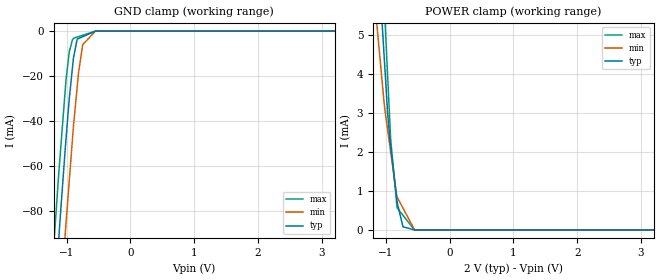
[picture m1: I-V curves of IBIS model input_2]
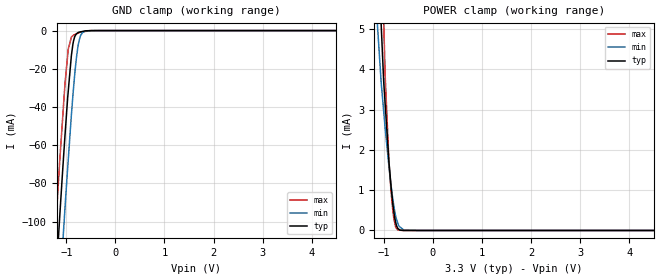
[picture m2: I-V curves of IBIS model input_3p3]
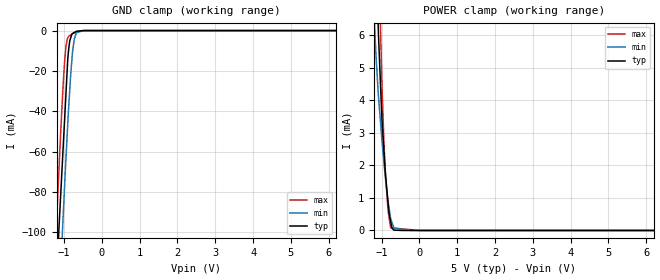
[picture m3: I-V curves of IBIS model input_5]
|Texas Instruments Incorporated
|16-Bit, Quad Channel, Ultralow Glitch, Voltage Output Digital to
|Analog Converter
|Marketing part#   Digital Voltage Range   Package-type   #pins
| DAC8555IPW   1.8V - 5.5V   TSSOP   16
| DAC8555IPWG4   1.8V - 5.5V   TSSOP   16
| DAC8555IPWR   1.8V - 5.5V   TSSOP   16
| DAC8555IPWRG4   1.8V - 5.5V   TSSOP   16
[IBIS Ver]   3.2
[File name]   dac8555.ibs
|SIMDE Ver   V3.0 - 201101 - RHL4 - Build 457
[File Rev]   1.0
[Date]   7/05/2011
[Source]
| Texas Instruments Incorporated.
| Analog-eLab Design Center, HPA
| 12500 TI Blvd
| Dallas, TX -75243
| e-mail: elab_ibis@list.ti.com
[Notes]   Revision History:
| Rev 1.0: 7/05/2011
| - Initial version of the model
| - Model generated from simulations in TISPICE
| - Model matched to SPICE simulation
| - C_comp although listed in numerical order of value are
|   obtained from varying PVT conditions. For PVT conditions for
|   each specific value refer the buffer description under
|   respective [Model]. IBIS model user is responsible for using
|   appropriate C_comp to simulate for Signal Integrity.
| - Model names with a trailing _2 contains the model for
|   2V [1.8V and 2.2V].
| - Model names with a trailing _3p3 contains the model for
|   3.3V [3.0V and 3.6V]. Model names with a trailing _5 contains
|   the model for 5.0V [4.5V and 5.5V].
[Disclaimer]
| This model is designed as an aid for customers of Texas Instruments.
| TI and its licensors and suppliers make no warranties, either expressed
| or implied, with respect to this  model, including the warranties of
| merchantability or fitness for a particular purpose. The model is
| provided solely on an "as is" basis. The entire risk as to its quality
| and performance is with the customer.
[Copyright]
 (C) Copyright 2011 Texas Instruments Incorporated.All rights reserved.
|   DAC8555
[Component]   DAC8555
[Manufacturer]   TI
[Package]   |16 TSSOP - PW package
|   typ   min   max
R_pkg   0.08290   0.07526   0.09084
L_pkg   2.48924nH   2.17582nH   2.84972nH
C_pkg   0.46616pF   0.44948pF   0.49354pF
[Pin]  signal_name   model_name   R_pin   L_pin   C_pin
1   VOUTA   TERM   0.08054   2.84007nH  0.49317pF
2   VOUTB   TERM   0.09081   2.45401nH  0.45118pF
3   VREFH   TERM   0.08088   2.27202nH  0.45822pF
4   AVDD   POWER   0.07498   2.16900nH  0.45240pF
5   VREFL   TERM   0.07526   2.17582nH  0.45462pF
6   GND   GND   0.03177   1.92365nH  0.50756pF
7   VOUTC   TERM   0.09084   2.46078nH  0.45336pF
8   VOUTD   TERM   0.08053   2.84799nH  0.49354pF
9   SYNC   INPUT   0.08056   2.84972nH  0.49331pF
10   SCLK   INPUT   0.08925   2.43251nH  0.44958pF
11   DIN   INPUT   0.08156   2.28822nH  0.45819pF
12   IOVDD   POWER   0.07619   2.19216nH  0.45412pF
13   RST   INPUT   0.07583   2.18360nH  0.45382pF
14   RSTSEL   INPUT   0.08162   2.28499nH  0.45822pF
15   ENABLE   INPUT   0.08934   2.42818nH  0.44948pF
16   LDAC   INPUT   0.08066   2.84222nH  0.49338pF
|   Model Selectors
[Model Selector] INPUT
input_2   2.0V digital input
input_3p3  3.3V digital input
input_5   5.0V digital input
[Model Selector] TERM
term_2   2V   nominal termination
term_3p3  3.3V nominal termination
term_5   5.0V nominal termination
[Model] term_2
Model_type Terminator
C_comp   1.0e-20F  1.0e-20F  1.0e-20F
|   typ   min   max
[Voltage Range]   2V   1.8V   2.2V
[POWER Clamp Reference]   2V   1.8V   2.2V
[GND Clamp Reference]   0V   0V   0V
|Ambient Temperature   25   105   -40
|Junction Temperature
[Temperature Range]   25   105   -40
[Model] term_3p3
Model_type Terminator
C_comp   1.0e-20F  1.0e-20F  1.0e-20F
|   typ   min   max
[Voltage Range]   3.3V   3.0V   3.6V
[POWER Clamp Reference]   3.3V   3.0V   3.6V
[GND Clamp Reference]   0V   0V   0V
|Ambient Temperature   25   105   -40
|Junction Temperature
[Temperature Range]   25   105   -40
[Model] term_5
Model_type Terminator
C_comp   1.0e-20F  1.0e-20F  1.0e-20F
|   typ   min   max
[Voltage Range]   5.0V   4.5V   5.5V
[POWER Clamp Reference]   5.0V   4.5V   5.5V
[GND Clamp Reference]   0V   0V   0V
|Ambient Temperature   25   105   -40
|Junction Temperature
[Temperature Range]   25   105   -40
| Models and submodels in the file (6): input_2 (Input), input_3p3 (Input), input_5 (Input), term_2 (Terminator), term_3p3 (Terminator), term_5 (Terminator)
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|   input_2 Model
[Model]   input_2
Model_type   Input
Vinl = 0.2
Vinh = 1.9
|   typ   min   max
|   (nom PVT)   (fast PVT)   (slow PVT)
|C_comp from frequency sweep method (F=50MHz)
|Average
|C_comp   1.219e-12   1.214e-12   1.231e-12
|C_comp from LC tank measurement(L=1nH)
|Average
|Resonant Frequency(Hz)   5.650e+09   5.970e+09   5.380e+09
C_comp   7.943e-13   7.114e-13   8.760e-13
| Where nom  PVT is Nominal Process, 2V, 25C
|Fast PVT is Strong Process,  2.2V, -40C
|Slow PVT is Weak Process,   1.8V, 105C
[Model Spec]
|Subparameter   typ   min   max
Vinh   1.9   1.71   2.09
Vinl   0.2   0.18   0.22
[Voltage Range]   2   1.8   2.2
|Ambient Temperature   25   105   -40
|Junction Temperature
[Temperature Range]   25   105   -40
[Power Clamp Reference]   2   1.8   2.2
[GND Clamp Reference]   0   0   0
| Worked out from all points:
|   GND clamp passes 1 mA (typ) near -0.63 V on its own axis
|   POWER clamp passes 1 mA (typ) near -0.84 V on its own axis
[GND Clamp]
|   Voltage   I(typ)   I(min)   I(max)
-2V       -477.6mA   -513.1mA   -450.5mA
-1.206V   -127mA     -166.3mA   -97.71mA
-1.124V   -93.3mA    -132.7mA   -64.03mA
-1.09V    -79.2mA    -118.6mA   -51.48mA
-1.024V   -53.78mA   -91.57mA   -27.33mA
-1.012V   -49.07mA   -86.77mA   -22.85mA
-959.2mV  -30.58mA   -67.17mA   -9.377mA
-891mV    -11.75mA   -42.04mA   -3.193mA
-834mV    -3.58mA    -24.9mA    -2.668mA
-747mV    -2.496mA   -6.029mA   -1.868mA
-549mV    -38.95uA   -67.57uA   -53.99uA
4V        0A         0A         0A
[POWER Clamp]
|   Voltage   I(typ)   I(min)   I(max)
-2V       49.4mA     36.45mA    63.1mA
-1.131V   7.955mA    5.115mA    11.35mA
-1.074V   5.746mA    4.111mA    8.39mA
-1.024V   4.418mA    3.23mA     6.018mA
-1.005V   3.917mA    2.976mA    5.142mA
-970mV    2.973mA    2.557mA    3.924mA
-924mV    2.14mA     2.013mA    2.34mA
-826.2mV  777uA      856.4uA    627.3uA
-822.8mV  729.6uA    845.9uA    567.7uA
-730mV    81.32uA    560.2uA    374.6uA
-549mV    127.1nA    3.062uA    12.93nA
4V        0A         0A         0A
|   input_3p3 Model
[Model]   input_3p3
Model_type   Input
Vinl = 0.99
Vinh = 2.31
|   typ   min   max
|   (nom PVT)   (fast PVT)   (slow PVT)
|C_comp from frequency sweep method (F=50MHz)
|Average
|C_comp   1.145e-12   1.058e-12   1.229e-12
|C_comp from LC tank measurement(L=1nH)
|Average
|Resonant Frequency(Hz)   5.770e+09   6.030e+09   5.540e+09
C_comp   7.616e-13   6.973e-13   8.261e-13
| Where nom  PVT is Nominal Process, 3.3V, 25C
|Fast PVT is Strong Process,  3.6V, -40C
|Slow PVT is Weak Process,   3V, 105C
[Model Spec]
|Subparameter   typ   min   max
Vinh   2.31   2.1   2.52
Vinl   0.99   0.9   1.08
[Voltage Range]   3.3   3   3.6
|Ambient Temperature   25   105   -40
|Junction Temperature
[Temperature Range]   25   105   -40
[Power Clamp Reference]   3.3   3   3.6
[GND Clamp Reference]   0   0   0
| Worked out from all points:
|   GND clamp passes 1 mA (typ) near -0.76 V on its own axis
|   POWER clamp passes 1 mA (typ) near -0.84 V on its own axis
[GND Clamp]
|   Voltage   I(typ)   I(min)   I(max)
-3.3V     -1.068A    -1.102A    -1.044A
-1.234V   -138.9mA   -179.1mA   -110.1mA
-1.138V   -98.64mA   -137.8mA   -69.42mA
-1.076V   -73.55mA   -112.5mA   -46.04mA
-1.03V    -55.64mA   -93.74mA   -28.57mA
-961.2mV  -31.76mA   -67.72mA   -9.751mA
-897.6mV  -13.13mA   -44.3mA    -3.486mA
-834.9mV  -3.649mA   -24.62mA   -2.132mA
-745.8mV  -874.7uA   -6.022mA   -1.167mA
-672mV    -472.3uA   -1.074mA   -721.6uA
-417mV    -13.81uA   -2.854uA   -1.605uA
6.6V      0A         0A         0A
[POWER Clamp]
|   Voltage   I(typ)   I(min)   I(max)
-3.3V     115.5mA    90.97mA    143.3mA
-1.158V   9.023mA    5.617mA    13.17mA
-1.096V   6.498mA    4.445mA    9.694mA
-1.051V   5.028mA    3.634mA    7.245mA
-1.003V   3.701mA    2.959mA    5.168mA
-972mV    3.116mA    2.521mA    3.817mA
-896.4mV  1.706mA    1.593mA    1.718mA
-874.8mV  1.4mA      1.356mA    1.317mA
-795.6mV  465.8uA    601.3uA    293.9uA
-712.8mV  45.75uA    172.5uA    11.65uA
-285mV    298.8nA    0A         0A
6.6V      0A         0A         0A
|   input_5 Model
[Model]   input_5
Model_type   Input
Vinl = 1.5
Vinh = 3.5
|   typ   min   max
|   (nom PVT)   (fast PVT)   (slow PVT)
|C_comp from frequency sweep method (F=50MHz)
|Average
|C_comp   1.036e-12   1.024e-12   1.068e-12
|C_comp from LC tank measurement(L=1nH)
|Average
|Resonant Frequency(Hz)   5.900e+09   6.120e+09   5.710e+09
C_comp   7.284e-13   6.770e-13   7.777e-13
| Where nom  PVT is Nominal Process, 5V, 25C
|Fast PVT is Strong Process,  5.5V, -40C
|Slow PVT is Weak Process,   4.5V, 105C
[Model Spec]
|Subparameter   typ   min   max
Vinh   3.5   3.15   3.85
Vinl   1.5   1.35   1.65
[Voltage Range]   5   4.5   5.5
|Ambient Temperature   25   105   -40
|Junction Temperature
[Temperature Range]   25   105   -40
[Power Clamp Reference]   5   4.5   5.5
[GND Clamp Reference]   0   0   0
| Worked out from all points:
|   GND clamp passes 1 mA (typ) near -0.74 V on its own axis
|   POWER clamp passes 1 mA (typ) near -0.84 V on its own axis
[GND Clamp]
|   Voltage   I(typ)   I(min)   I(max)
-5V       -1.845A    -1.876A    -1.825A
-1.206V   -127.5mA   -166.3mA   -98.22mA
-1.14V    -99.51mA   -138.9mA   -70.55mA
-1.071V   -74.66mA   -110.3mA   -43.57mA
-1.028V   -59.35mA   -93.57mA   -28.2mA
-951.5mV  -31.62mA   -63.85mA   -8.06mA
-905mV    -14.87mA   -46.93mA   -3.728mA
-875mV    -8.588mA   -36.89mA   -2.79mA
-774mV    -1.407mA   -10.15mA   -1.62mA
-729mV    -937.2uA   -4.088mA   -1.124mA
-675mV    -373.2uA   -1.153mA   -583.8uA
10V       0A         0A         0A
[POWER Clamp]
|   Voltage   I(typ)   I(min)   I(max)
-5V       202.4mA    162.9mA    248.2mA
-1.21V    11.13mA    6.945mA    15.8mA
-1.152V   8.685mA    5.481mA    12.53mA
-1.089V   6.284mA    4.24mA     9.145mA
-1.056V   5.268mA    3.733mA    7.48mA
-990mV    3.396mA    2.758mA    4.505mA
-940.5mV  2.488mA    2.12mA     2.788mA
-907.5mV  1.882mA    1.724mA    1.952mA
-841.5mV  1.009mA    1.003mA    805.5uA
-759mV    269.6uA    356.8uA    84.33uA
-670mV    9.915uA    71.14uA    74.44uA
10V       0A         0A         0A
